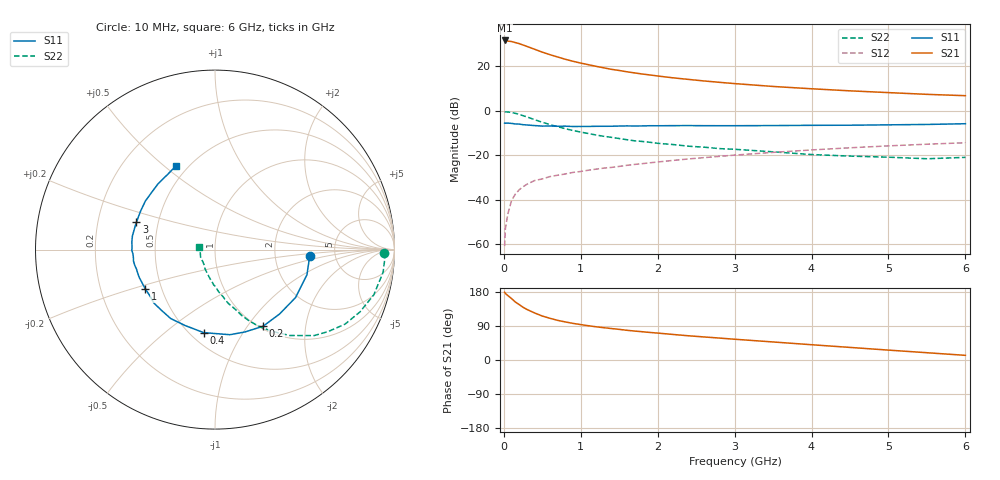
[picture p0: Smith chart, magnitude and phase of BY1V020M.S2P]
! SIEMENS Small Signal Semiconductors
! BFY420
! Si NPN RF SIEGET Grounded Emitter Transistor in MICRO-X
! VCE = 1 V  IC = 20 mA
! Common Emitter S-Parameters:  October  1996
# GHz  S  MA  R  50
!  f  S11  S21  S12  S22
! GHz  MAG  ANG  MAG  ANG  MAG  ANG  MAG  ANG
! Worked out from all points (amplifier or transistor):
!   36 points, 10 MHz to 6 GHz, reference 50 ohm
!   highest |S21| = 31.7 dB at 10 MHz (marker M1)
!   |S21| within 3 dB of that: start of sweep to 324.9 MHz
!   unconditionally stable (mu >= 1): 1.762 GHz to end of sweep
!   at 250 MHz: K = 0.31, MSG = 31.9 dB, |S12| = -34.2 dB
!   at 1.4 GHz: K = 0.94, MSG = 22.1 dB, |S12| = -25.4 dB
!   at 6 GHz: K = 1.09, MAG = 8.8 dB, |S12| = -14.4 dB
!   S11 on the Smith chart (normalised r, x): 10 MHz: 3.23, -0.32; 200 MHz: 1.04, -1.19; 400 MHz: 0.58, -0.69; 1 GHz: 0.41, -0.22; 3 GHz: 0.38, +0.15; 6 GHz: 0.43, +0.55
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0.01  0.5313 -3.8  38.48 178.7  0.0009 112.1  0.9431 -1.1
0.02  0.5276 -6.6  38.13 175.7  0.0022 83.5  0.9479 -2.7
0.1  0.5223 -30.8  36.39 162.1  0.0096 76.9  0.92 -15.9
0.15  0.508 -45.0  34.46 153.0  0.0134 72.2  0.8789 -23.3
0.2  0.5041 -57.9  32.66 146.2  0.0168 69.1  0.8352 -29.8
0.25  0.4883 -70.0  30.39 139.1  0.0196 64.4  0.7794 -35.8
0.3  0.4814 -80.1  28.26 133.4  0.0223 62.0  0.7316 -40.9
0.4  0.4668 -97.8  24.38 124.1  0.027 57.9  0.6341 -49.0
0.5  0.4546 -111.6  20.98 116.0  0.0294 55.6  0.5539 -55.2
0.6  0.4566 -122.7  18.4 110.0  0.0332 54.0  0.4911 -60.3
0.7  0.451 -131.4  16.33 104.6  0.0356 54.1  0.4403 -64.4
0.8  0.4524 -138.8  14.5 100.4  0.038 52.9  0.3963 -67.9
1  0.4459 -150.3  11.89 93.4  0.0432 53.3  0.333 -73.1
1.1  0.4464 -155.3  10.94 90.4  0.0462 53.6  0.3089 -76.1
1.4  0.4508 -166.1  8.613 83.0  0.0534 54.1  0.2533 -82.3
1.6  0.4586 -172.1  7.581 78.4  0.0595 53.3  0.2244 -86.6
2.2  0.4653 174.7  5.542 67.4  0.0767 51.9  0.1747 -97.0
3  0.4635 160.7  4.112 54.8  0.101 47.8  0.1365 -109.2
3.5  0.4668 152.8  3.546 47.6  0.1163 44.5  0.1197 -117.8
4.5  0.4756 137.9  2.825 33.2  0.1476 35.8  0.0959 -135.0
5.5  0.4948 122.4  2.355 19.2  0.1777 26.0  0.0836 -169.6
6  0.5137 115.2  2.198 12.3  0.1916 21.0  0.0898 171.0
